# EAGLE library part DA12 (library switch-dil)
DIL/CODE SWITCH
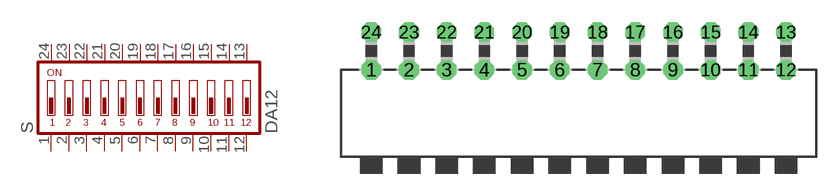
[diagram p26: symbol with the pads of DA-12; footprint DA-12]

Designator prefix S

## DA12 (OC_FARNELL: 1255232; OC_NEWARK: unknown)  [DA-12]
1  1  pas
2  2  pas
3  3  pas
4  4  pas
5  5  pas
6  6  pas
7  7  pas
8  8  pas
9  9  pas
10  10  pas
11  11  pas
12  12  pas
13  13  pas
14  14  pas
15  15  pas
16  16  pas
17  17  pas
18  18  pas
19  19  pas
20  20  pas
21  21  pas
22  22  pas
23  23  pas
24  24  pas

## Footprint DA-12 (pad centres in mm)
DIL/CODE SWITCH Mors distributor Buerklin, 17G598
drill 0.813 octagon: 1 -13.97,-1.27; 2 -11.43,-1.27; 3 -8.89,-1.27; 4 -6.35,-1.27; 5 -3.81,-1.27; 6 -1.27,-1.27; 7 1.27,-1.27; 8 3.81,-1.27; 9 6.35,-1.27; 10 8.89,-1.27; 11 11.43,-1.27; 12 13.97,-1.27; 13 13.97,1.27; 14 11.43,1.27; 15 8.89,1.27; 16 6.35,1.27; 17 3.81,1.27; 18 1.27,1.27; 19 -1.27,1.27; 20 -3.81,1.27; 21 -6.35,1.27; 22 -8.89,1.27; 23 -11.43,1.27; 24 -13.97,1.27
